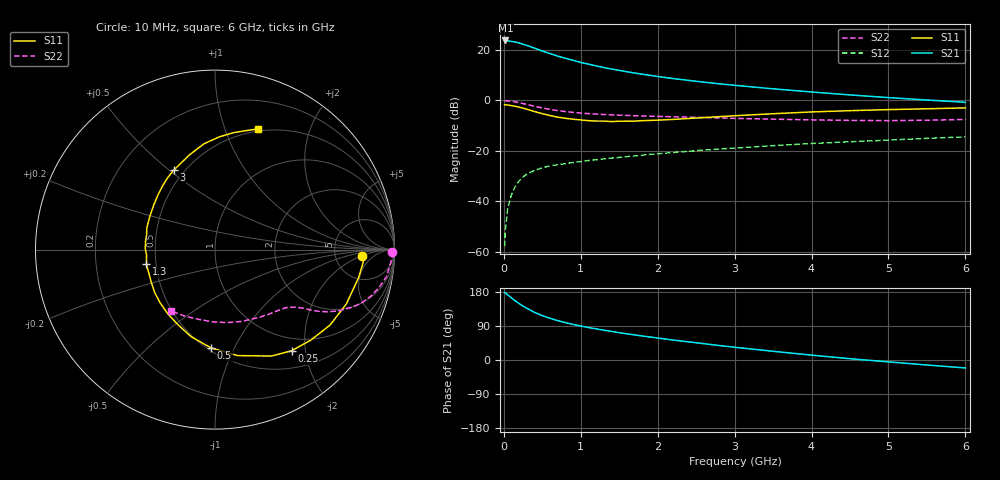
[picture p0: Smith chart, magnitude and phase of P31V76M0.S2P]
! SIEMENS Small Signal Semiconductors
! BFP181
! Si NPN RF Bipolar Junction Transistor in SOT143
! VCE = 1.75 V  IC = 6 mA
! Common Emitter S-Parameters:  March  1996
# GHz  S  MA  R  50
!  f  S11  S21  S12  S22
! GHz  MAG  ANG  MAG  ANG  MAG  ANG  MAG  ANG
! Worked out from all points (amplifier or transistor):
!   36 points, 10 MHz to 6 GHz, reference 50 ohm
!   highest |S21| = 23.8 dB at 20 MHz (marker M1)
!   |S21| within 3 dB of that: start of sweep to 395.4 MHz
!   unconditionally stable (mu >= 1): 1.39 GHz to end of sweep
!   at 250 MHz: K = 0.25, MSG = 26.3 dB, |S12| = -30.3 dB
!   at 1.4 GHz: K = 1.00, MAG = 17.3 dB, |S12| = -22.8 dB
!   at 6 GHz: K = 1.05, MAG = 5.5 dB, |S12| = -14.4 dB
!   S11 on the Smith chart (normalised r, x): 10 MHz: 9.65, -2.02; 250 MHz: 0.77, -1.74; 500 MHz: 0.52, -0.82; 1.3 GHz: 0.44, -0.09; 3 GHz: 0.44, +0.52; 6 GHz: 0.48, +1.31
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0.01  0.8195 -2.4  15.31 178.5  0.0013 86.6  0.9873 -0.8
0.02  0.829 -4.8  15.46 177.1  0.0028 89.4  0.989 -1.9
0.05  0.8151 -11.1  15.28 171.8  0.0073 86.8  0.9806 -4.6
0.15  0.7667 -33.2  14.41 155.8  0.0202 72.0  0.9364 -13.2
0.2  0.7347 -43.3  13.78 148.8  0.0256 67.5  0.9052 -16.8
0.25  0.7068 -52.9  12.98 142.1  0.0306 64.5  0.8699 -19.9
0.3  0.6712 -62.1  12.34 136.4  0.0348 60.7  0.834 -22.5
0.4  0.6034 -78.1  10.88 125.6  0.0412 54.7  0.7668 -26.5
0.5  0.5484 -92.2  9.535 117.1  0.0463 49.7  0.7122 -29.1
0.6  0.5035 -105.2  8.52 110.1  0.0508 47.2  0.6669 -31.0
0.7  0.4674 -116.0  7.554 103.9  0.0534 45.2  0.6314 -32.2
0.8  0.4437 -126.5  6.863 98.6  0.056 44.2  0.6034 -33.1
0.9  0.4258 -136.0  6.23 94.0  0.0592 43.3  0.5807 -34.0
1.1  0.3985 -153.2  5.248 85.6  0.0647 42.3  0.5494 -35.7
1.3  0.3907 -167.9  4.486 78.7  0.0695 41.2  0.5279 -37.5
1.7  0.39 167.6  3.5 66.2  0.0797 41.0  0.4995 -41.4
2.2  0.4218 144.1  2.721 52.6  0.0932 39.7  0.4759 -47.7
3  0.4985 117.5  2.001 33.7  0.1144 36.1  0.4419 -60.2
3.5  0.5467 105.1  1.702 23.0  0.1274 33.2  0.4269 -69.6
4.5  0.6287 87.8  1.289 3.4  0.1522 26.5  0.4034 -91.3
5.5  0.6848 75.4  1.022 -13.2  0.1778 20.4  0.4072 -114.3
6  0.7142 70.3  0.921 -21.0  0.1904 16.4  0.4211 -125.9
